(* Logix 5000 AddOnInstructionDefinition export Banner_WLS_Param_v4; software revision 33.00; part 2 of 3 *)
(* tags used below, declared in another part *)
   WLS : Banner_WLS_v4;
   Port_Data : Banner_IOL_Port_v4;
   Port : INT;   // Port Number that device is plugged into.
   Type : SINT;   // 0 = WLS27, 1 = WLS15, 2 = WLF
   Local_Control : DINT;
   Command_Being_Processed : BOOL;
   Update_Archive : BOOL;
   Index_Write_Inprocess : DINT;
   Index_Write_Control : DINT;
   Inprocess_Index : DINT;
   IndexR : DINT;   // Index keeping track of Reads in an array.
   S_Index : DINT;
   IndexW : DINT;   // Index keeping track of Writes in an array.
   LT_Index : DINT;
   IndexW2 : DINT;
   G_Index : DINT;
   IndexW3 : DINT;
(* Banner_WLS_Param_v4, continued *)

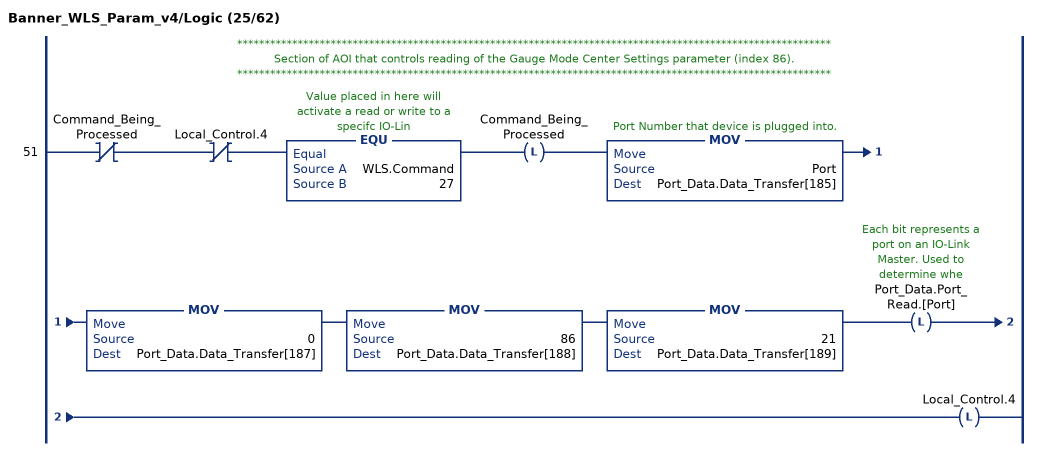
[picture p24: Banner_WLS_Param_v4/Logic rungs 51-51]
   // ************************************************************************************************************
   // Section of AOI that controls reading of the Gauge Mode Center Settings parameter (index 86).
   // ************************************************************************************************************
   51: XIO(Command_Being_Processed)XIO(Local_Control.4)EQU(WLS.Command,27)OTL(Command_Being_Processed)MOV(Port,Port_Data.Data_Transfer[185])MOV(0,Port_Data.Data_Transfer[187])MOV(86,Port_Data.Data_Transfer[188])MOV(21,Port_Data.Data_Transfer[189])OTL(Port_Data.Port_Read.[Port])OTL(Local_Control.4);
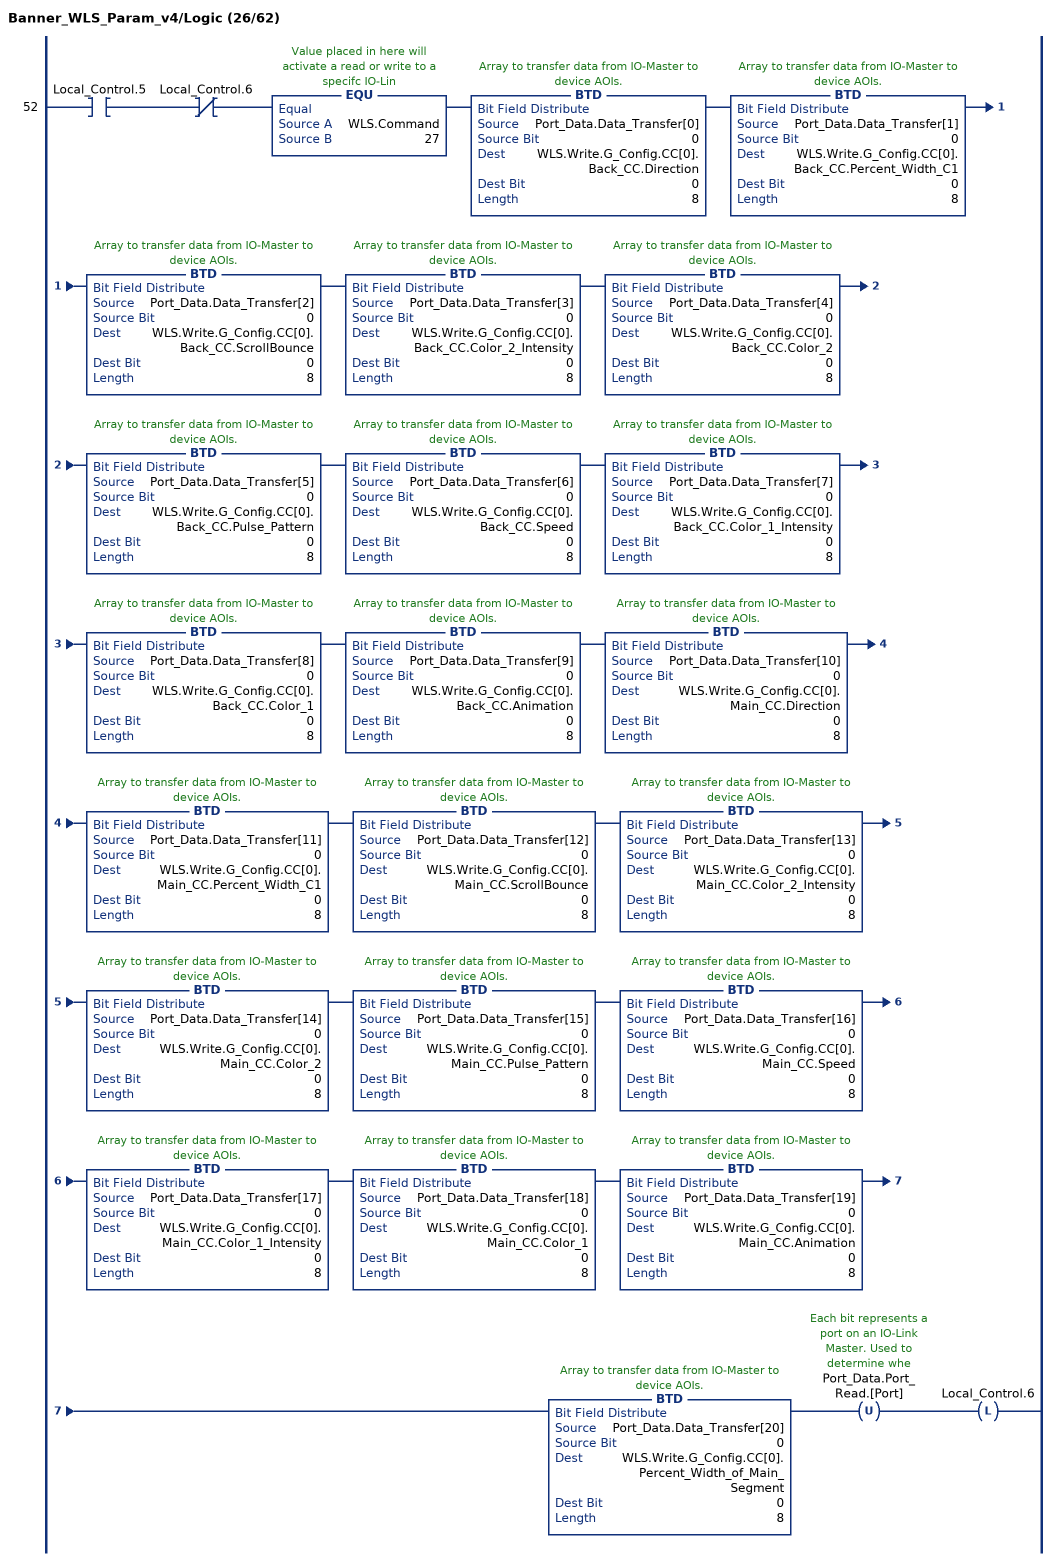
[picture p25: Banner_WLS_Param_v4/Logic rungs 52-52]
   52: XIC(Local_Control.5)XIO(Local_Control.6)EQU(WLS.Command,27)BTD(Port_Data.Data_Transfer[0],0,WLS.Write.G_Config.CC[0].Back_CC.Direction,0,8)BTD(Port_Data.Data_Transfer[1],0,WLS.Write.G_Config.CC[0].Back_CC.Percent_Width_C1,0,8)BTD(Port_Data.Data_Transfer[2],0,WLS.Write.G_Config.CC[0].Back_CC.ScrollBounce,0,8)BTD(Port_Data.Data_Transfer[3],0,WLS.Write.G_Config.CC[0].Back_CC.Color_2_Intensity,0,8)BTD(Port_Data.Data_Transfer[4],0,WLS.Write.G_Config.CC[0].Back_CC.Color_2,0,8)BTD(Port_Data.Data_Transfer[5],0,WLS.Write.G_Config.CC[0].Back_CC.Pulse_Pattern,0,8)BTD(Port_Data.Data_Transfer[6],0,WLS.Write.G_Config.CC[0].Back_CC.Speed,0,8)BTD(Port_Data.Data_Transfer[7],0,WLS.Write.G_Config.CC[0].Back_CC.Color_1_Intensity,0,8)BTD(Port_Data.Data_Transfer[8],0,WLS.Write.G_Config.CC[0].Back_CC.Color_1,0,8)BTD(Port_Data.Data_Transfer[9],0,WLS.Write.G_Config.CC[0].Back_CC.Animation,0,8)BTD(Port_Data.Data_Transfer[10],0,WLS.Write.G_Config.CC[0].Main_CC.Direction,0,8)BTD(Port_Data.Data_Transfer[11],0,WLS.Write.G_Config.CC[0].Main_CC.Percent_Width_C1,0,8)BTD(Port_Data.Data_Transfer[12],0,WLS.Write.G_Config.CC[0].Main_CC.ScrollBounce,0,8)BTD(Port_Data.Data_Transfer[13],0,WLS.Write.G_Config.CC[0].Main_CC.Color_2_Intensity,0,8)BTD(Port_Data.Data_Transfer[14],0,WLS.Write.G_Config.CC[0].Main_CC.Color_2,0,8)BTD(Port_Data.Data_Transfer[15],0,WLS.Write.G_Config.CC[0].Main_CC.Pulse_Pattern,0,8)BTD(Port_Data.Data_Transfer[16],0,WLS.Write.G_Config.CC[0].Main_CC.Speed,0,8)BTD(Port_Data.Data_Transfer[17],0,WLS.Write.G_Config.CC[0].Main_CC.Color_1_Intensity,0,8)BTD(Port_Data.Data_Transfer[18],0,WLS.Write.G_Config.CC[0].Main_CC.Color_1,0,8)BTD(Port_Data.Data_Transfer[19],0,WLS.Write.G_Config.CC[0].Main_CC.Animation,0,8)BTD(Port_Data.Data_Transfer[20],0,WLS.Write.G_Config.CC[0].Percent_Width_of_Main_Segment,0,8)OTU(Port_Data.Port_Read.[Port])OTL(Local_Control.6);
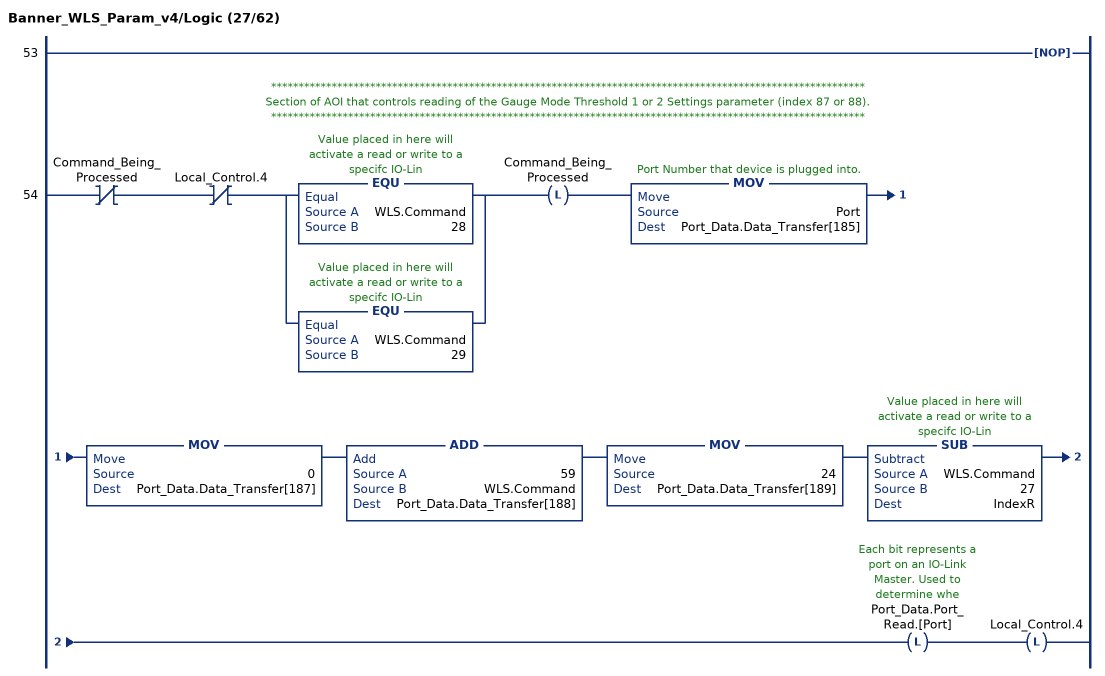
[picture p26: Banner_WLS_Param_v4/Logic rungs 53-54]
   53: NOP();
   // ************************************************************************************************************
   // Section of AOI that controls reading of the Gauge Mode Threshold 1 or 2 Settings parameter (index 87 or 88).
   // ************************************************************************************************************
   54: XIO(Command_Being_Processed)XIO(Local_Control.4)[EQU(WLS.Command,28) ,EQU(WLS.Command,29) ]OTL(Command_Being_Processed)MOV(Port,Port_Data.Data_Transfer[185])MOV(0,Port_Data.Data_Transfer[187])ADD(59,WLS.Command,Port_Data.Data_Transfer[188])MOV(24,Port_Data.Data_Transfer[189])SUB(WLS.Command,27,IndexR)OTL(Port_Data.Port_Read.[Port])OTL(Local_Control.4);
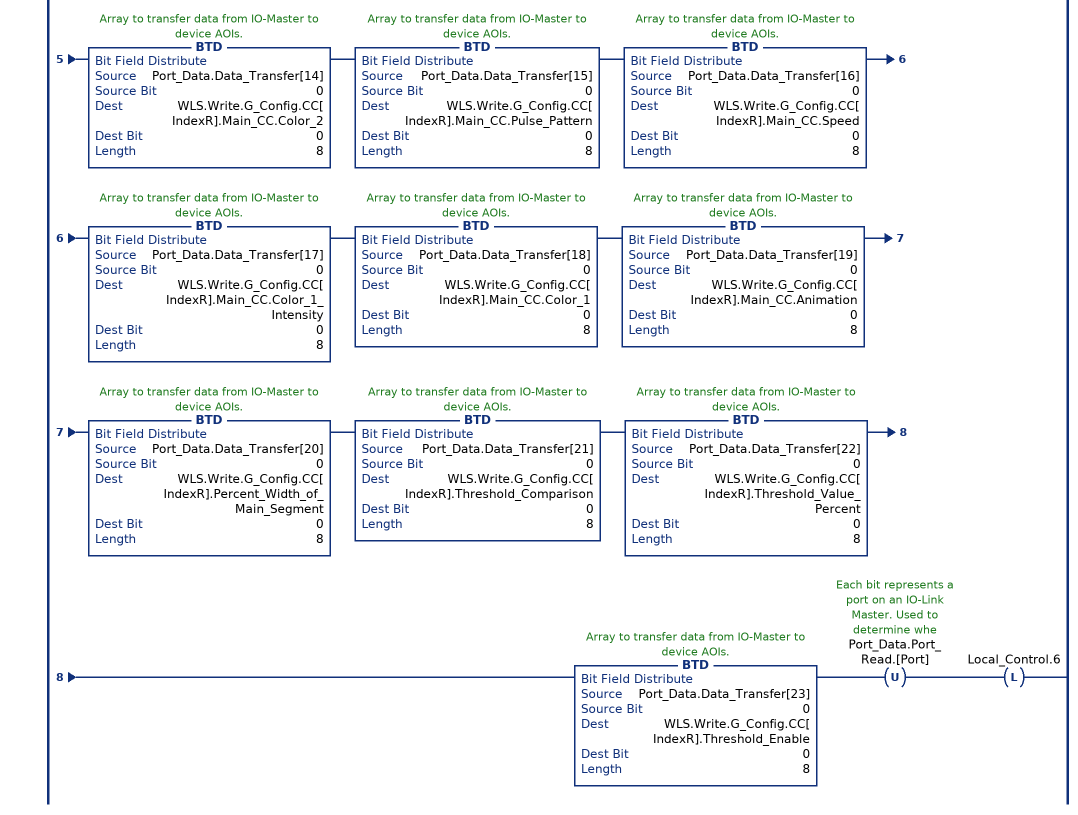
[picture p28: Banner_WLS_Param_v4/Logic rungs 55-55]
   55: XIC(Local_Control.5)XIO(Local_Control.6)[EQU(WLS.Command,28) ,EQU(WLS.Command,29) ]BTD(Port_Data.Data_Transfer[0],0,WLS.Write.G_Config.CC[IndexR].Back_CC.Direction,0,8)BTD(Port_Data.Data_Transfer[1],0,WLS.Write.G_Config.CC[IndexR].Back_CC.Percent_Width_C1,0,8)BTD(Port_Data.Data_Transfer[2],0,WLS.Write.G_Config.CC[IndexR].Back_CC.ScrollBounce,0,8)BTD(Port_Data.Data_Transfer[3],0,WLS.Write.G_Config.CC[IndexR].Back_CC.Color_2_Intensity,0,8)BTD(Port_Data.Data_Transfer[4],0,WLS.Write.G_Config.CC[IndexR].Back_CC.Color_2,0,8)BTD(Port_Data.Data_Transfer[5],0,WLS.Write.G_Config.CC[IndexR].Back_CC.Pulse_Pattern,0,8)BTD(Port_Data.Data_Transfer[6],0,WLS.Write.G_Config.CC[IndexR].Back_CC.Speed,0,8)BTD(Port_Data.Data_Transfer[7],0,WLS.Write.G_Config.CC[IndexR].Back_CC.Color_1_Intensity,0,8)BTD(Port_Data.Data_Transfer[8],0,WLS.Write.G_Config.CC[IndexR].Back_CC.Color_1,0,8)BTD(Port_Data.Data_Transfer[9],0,WLS.Write.G_Config.CC[IndexR].Back_CC.Animation,0,8)BTD(Port_Data.Data_Transfer[10],0,WLS.Write.G_Config.CC[IndexR].Main_CC.Direction,0,8)BTD(Port_Data.Data_Transfer[11],0,WLS.Write.G_Config.CC[IndexR].Main_CC.Percent_Width_C1,0,8)BTD(Port_Data.Data_Transfer[12],0,WLS.Write.G_Config.CC[IndexR].Main_CC.ScrollBounce,0,8)BTD(Port_Data.Data_Transfer[13],0,WLS.Write.G_Config.CC[IndexR].Main_CC.Color_2_Intensity,0,8)BTD(Port_Data.Data_Transfer[14],0,WLS.Write.G_Config.CC[IndexR].Main_CC.Color_2,0,8)BTD(Port_Data.Data_Transfer[15],0,WLS.Write.G_Config.CC[IndexR].Main_CC.Pulse_Pattern,0,8)BTD(Port_Data.Data_Transfer[16],0,WLS.Write.G_Config.CC[IndexR].Main_CC.Speed,0,8)BTD(Port_Data.Data_Transfer[17],0,WLS.Write.G_Config.CC[IndexR].Main_CC.Color_1_Intensity,0,8)BTD(Port_Data.Data_Transfer[18],0,WLS.Write.G_Config.CC[IndexR].Main_CC.Color_1,0,8)BTD(Port_Data.Data_Transfer[19],0,WLS.Write.G_Config.CC[IndexR].Main_CC.Animation,0,8)BTD(Port_Data.Data_Transfer[20],0,WLS.Write.G_Config.CC[IndexR].Percent_Width_of_Main_Segment,0,8)BTD(Port_Data.Data_Transfer[21],0,WLS.Write.G_Config.CC[IndexR].Threshold_Comparison,0,8)BTD(Port_Data.Data_Transfer[22],0,WLS.Write.G_Config.CC[IndexR].Threshold_Value_Percent,0,8)BTD(Port_Data.Data_Transfer[23],0,WLS.Write.G_Config.CC[IndexR].Threshold_Enable,0,8)OTU(Port_Data.Port_Read.[Port])OTL(Local_Control.6);
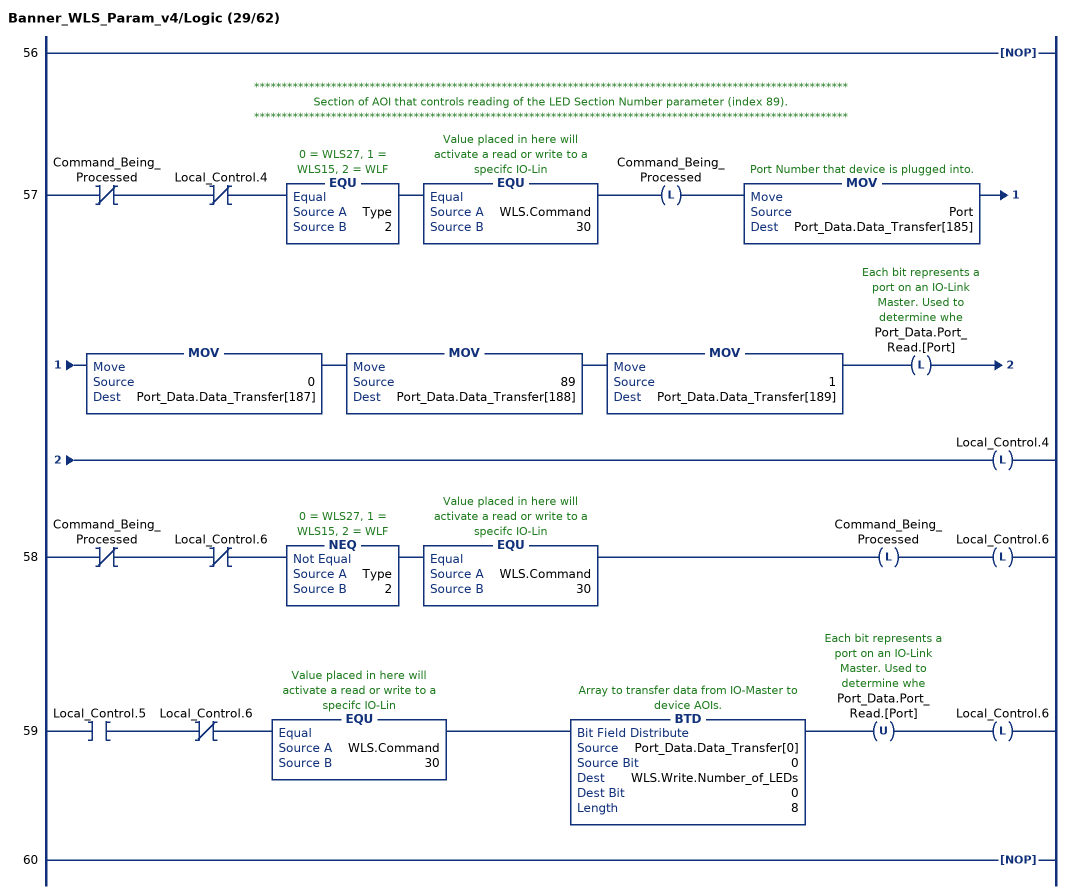
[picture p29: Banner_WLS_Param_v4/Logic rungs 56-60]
   56: NOP();
   // ************************************************************************************************************
   // Section of AOI that controls reading of the LED Section Number parameter (index 89).
   // ************************************************************************************************************
   57: XIO(Command_Being_Processed)XIO(Local_Control.4)EQU(Type,2)EQU(WLS.Command,30)OTL(Command_Being_Processed)MOV(Port,Port_Data.Data_Transfer[185])MOV(0,Port_Data.Data_Transfer[187])MOV(89,Port_Data.Data_Transfer[188])MOV(1,Port_Data.Data_Transfer[189])OTL(Port_Data.Port_Read.[Port])OTL(Local_Control.4);
   58: XIO(Command_Being_Processed)XIO(Local_Control.6)NEQ(Type,2)EQU(WLS.Command,30)OTL(Command_Being_Processed)OTL(Local_Control.6);
   59: XIC(Local_Control.5)XIO(Local_Control.6)EQU(WLS.Command,30)BTD(Port_Data.Data_Transfer[0],0,WLS.Write.Number_of_LEDs,0,8)OTU(Port_Data.Port_Read.[Port])OTL(Local_Control.6);
   60: NOP();
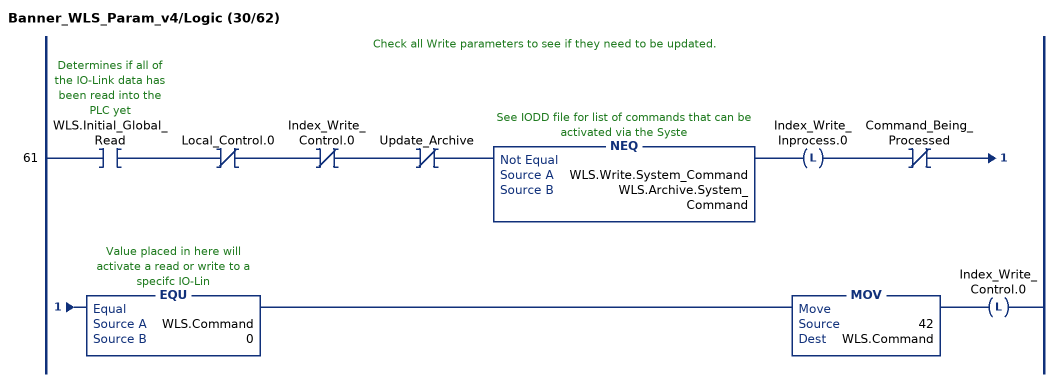
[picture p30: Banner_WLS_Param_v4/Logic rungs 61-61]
   // Check all Write parameters to see if they need to be updated.
   61: XIC(WLS.Initial_Global_Read)XIO(Local_Control.0)XIO(Index_Write_Control.0)XIO(Update_Archive)NEQ(WLS.Write.System_Command,WLS.Archive.System_Command)OTL(Index_Write_Inprocess.0)XIO(Command_Being_Processed)EQU(WLS.Command,0)MOV(42,WLS.Command)OTL(Index_Write_Control.0);
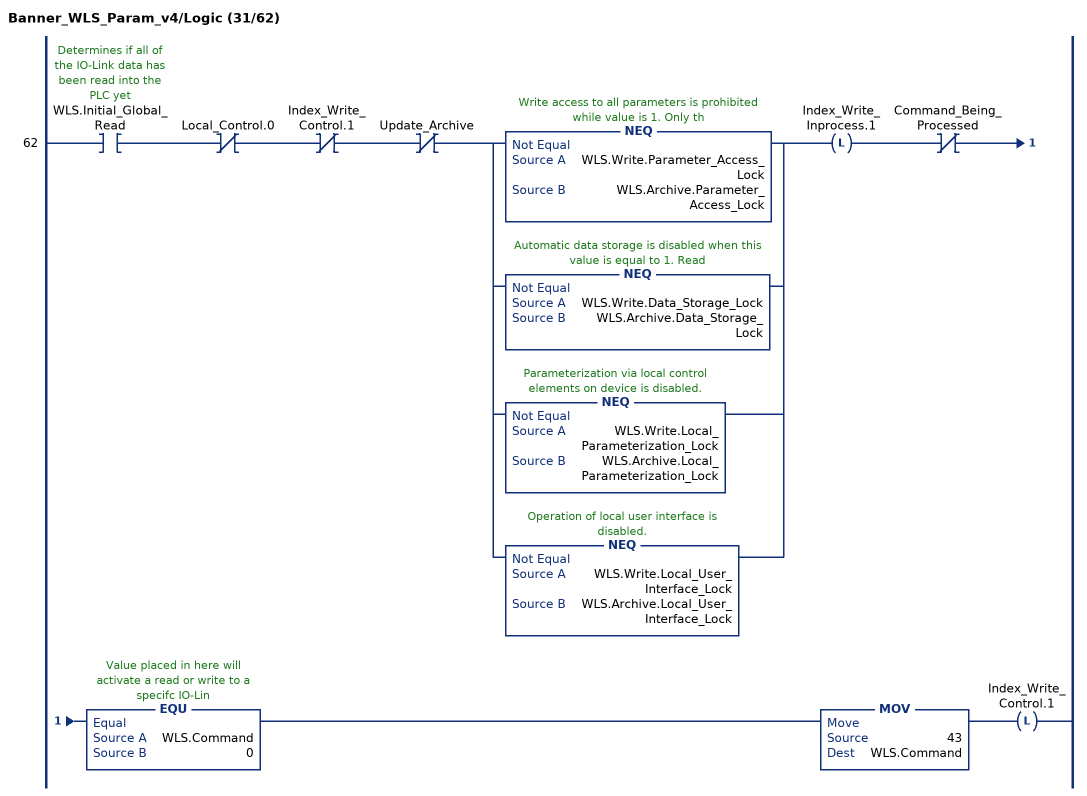
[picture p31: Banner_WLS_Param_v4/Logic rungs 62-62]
   62: XIC(WLS.Initial_Global_Read)XIO(Local_Control.0)XIO(Index_Write_Control.1)XIO(Update_Archive)[NEQ(WLS.Write.Parameter_Access_Lock,WLS.Archive.Parameter_Access_Lock) ,NEQ(WLS.Write.Data_Storage_Lock,WLS.Archive.Data_Storage_Lock) ,NEQ(WLS.Write.Local_Parameterization_Lock,WLS.Archive.Local_Parameterization_Lock) ,NEQ(WLS.Write.Local_User_Interface_Lock,WLS.Archive.Local_User_Interface_Lock) ]OTL(Index_Write_Inprocess.1)XIO(Command_Being_Processed)EQU(WLS.Command,0)MOV(43,WLS.Command)OTL(Index_Write_Control.1);
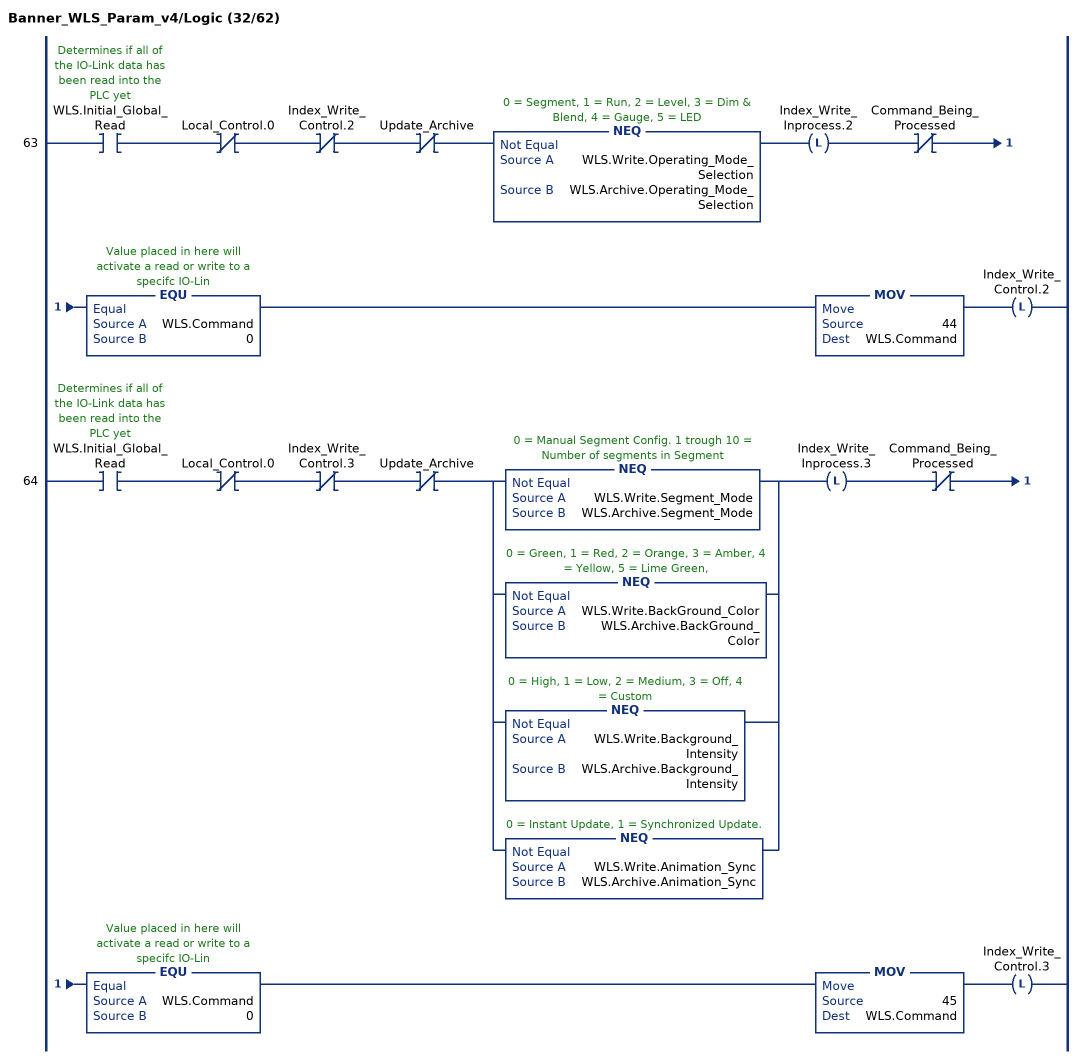
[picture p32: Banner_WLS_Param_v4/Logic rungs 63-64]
   63: XIC(WLS.Initial_Global_Read)XIO(Local_Control.0)XIO(Index_Write_Control.2)XIO(Update_Archive)NEQ(WLS.Write.Operating_Mode_Selection,WLS.Archive.Operating_Mode_Selection)OTL(Index_Write_Inprocess.2)XIO(Command_Being_Processed)EQU(WLS.Command,0)MOV(44,WLS.Command)OTL(Index_Write_Control.2);
   64: XIC(WLS.Initial_Global_Read)XIO(Local_Control.0)XIO(Index_Write_Control.3)XIO(Update_Archive)[NEQ(WLS.Write.Segment_Mode,WLS.Archive.Segment_Mode) ,NEQ(WLS.Write.BackGround_Color,WLS.Archive.BackGround_Color) ,NEQ(WLS.Write.Background_Intensity,WLS.Archive.Background_Intensity) ,NEQ(WLS.Write.Animation_Sync,WLS.Archive.Animation_Sync) ]OTL(Index_Write_Inprocess.3)XIO(Command_Being_Processed)EQU(WLS.Command,0)MOV(45,WLS.Command)OTL(Index_Write_Control.3);
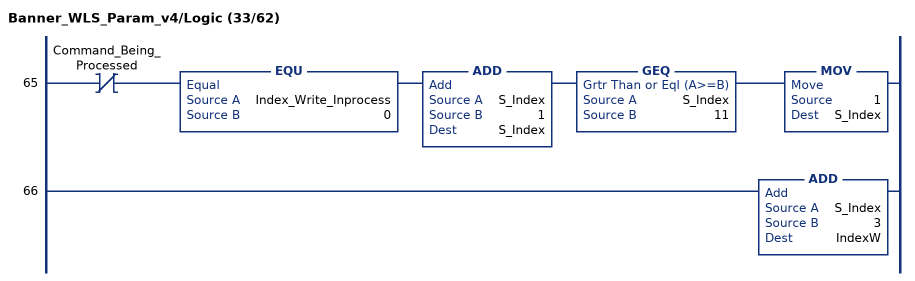
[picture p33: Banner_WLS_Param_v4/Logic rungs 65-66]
   65: XIO(Command_Being_Processed)EQU(Index_Write_Inprocess,0)ADD(S_Index,1,S_Index)GEQ(S_Index,11)MOV(1,S_Index);
   66: ADD(S_Index,3,IndexW);
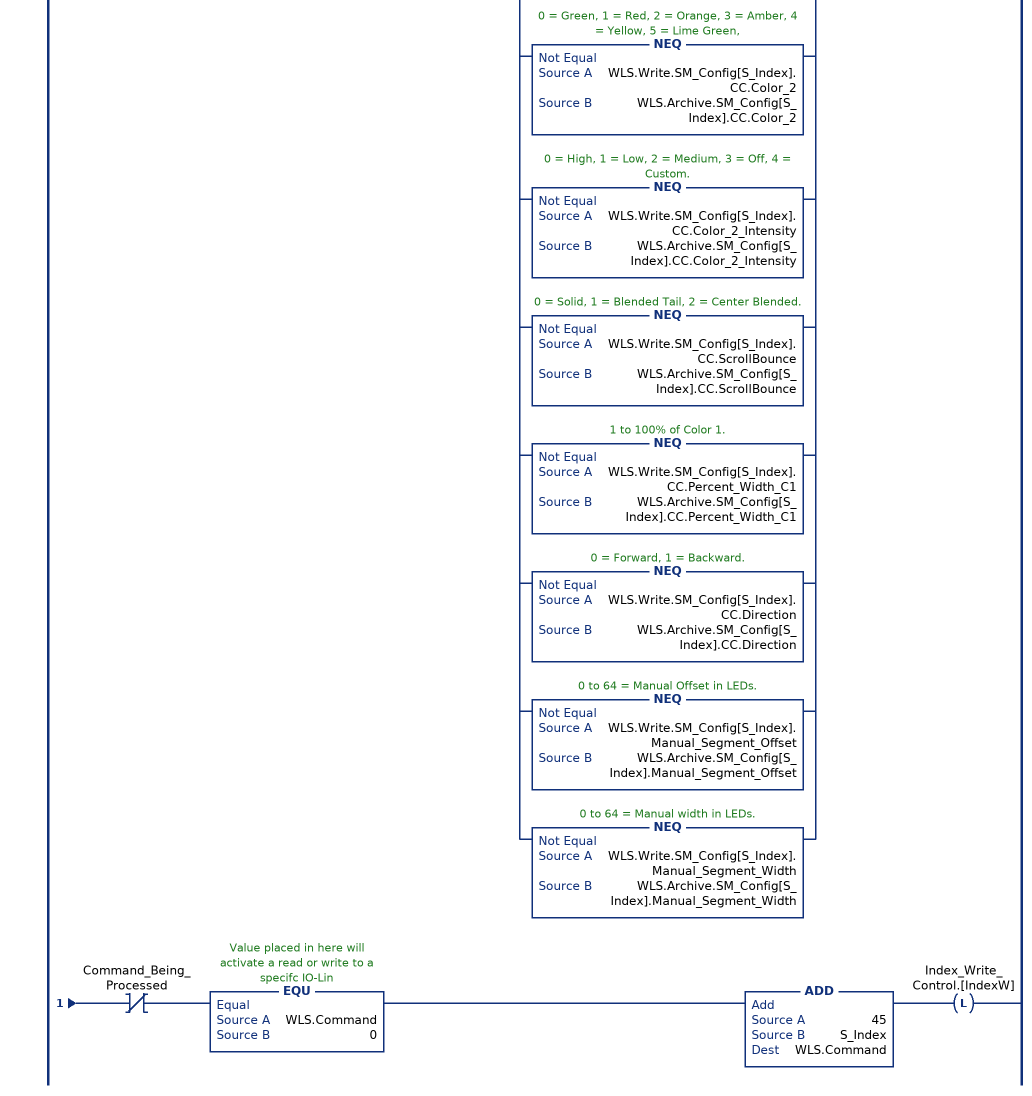
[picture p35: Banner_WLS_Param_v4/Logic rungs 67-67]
   67: XIC(WLS.Initial_Global_Read)XIO(Local_Control.0)XIO(Index_Write_Control.[IndexW])XIO(Update_Archive)[NEQ(WLS.Write.SM_Config[S_Index].Basic_Color,WLS.Archive.SM_Config[S_Index].Basic_Color) ,NEQ(WLS.Write.SM_Config[S_Index].Basic_Flash_Rate,WLS.Archive.SM_Config[S_Index].Basic_Flash_Rate) ,NEQ(WLS.Write.SM_Config[S_Index].CC.Animation,WLS.Archive.SM_Config[S_Index].CC.Animation) ,NEQ(WLS.Write.SM_Config[S_Index].CC.Color_1,WLS.Archive.SM_Config[S_Index].CC.Color_1) ,NEQ(WLS.Write.SM_Config[S_Index].CC.Color_1_Intensity,WLS.Archive.SM_Config[S_Index].CC.Color_1_Intensity) ,NEQ(WLS.Write.SM_Config[S_Index].CC.Speed,WLS.Archive.SM_Config[S_Index].CC.Speed) ,NEQ(WLS.Write.SM_Config[S_Index].CC.Pulse_Pattern,WLS.Archive.SM_Config[S_Index].CC.Pulse_Pattern) ,NEQ(WLS.Write.SM_Config[S_Index].CC.Color_2,WLS.Archive.SM_Config[S_Index].CC.Color_2) ,NEQ(WLS.Write.SM_Config[S_Index].CC.Color_2_Intensity,WLS.Archive.SM_Config[S_Index].CC.Color_2_Intensity) ,NEQ(WLS.Write.SM_Config[S_Index].CC.ScrollBounce,WLS.Archive.SM_Config[S_Index].CC.ScrollBounce) ,NEQ(WLS.Write.SM_Config[S_Index].CC.Percent_Width_C1,WLS.Archive.SM_Config[S_Index].CC.Percent_Width_C1) ,NEQ(WLS.Write.SM_Config[S_Index].CC.Direction,WLS.Archive.SM_Config[S_Index].CC.Direction) ,NEQ(WLS.Write.SM_Config[S_Index].Manual_Segment_Offset,WLS.Archive.SM_Config[S_Index].Manual_Segment_Offset) ,NEQ(WLS.Write.SM_Config[S_Index].Manual_Segment_Width,WLS.Archive.SM_Config[S_Index].Manual_Segment_Width) ]OTL(Index_Write_Inprocess.[IndexW])XIO(Command_Being_Processed)EQU(WLS.Command,0)ADD(45,S_Index,WLS.Command)OTL(Index_Write_Control.[IndexW]);
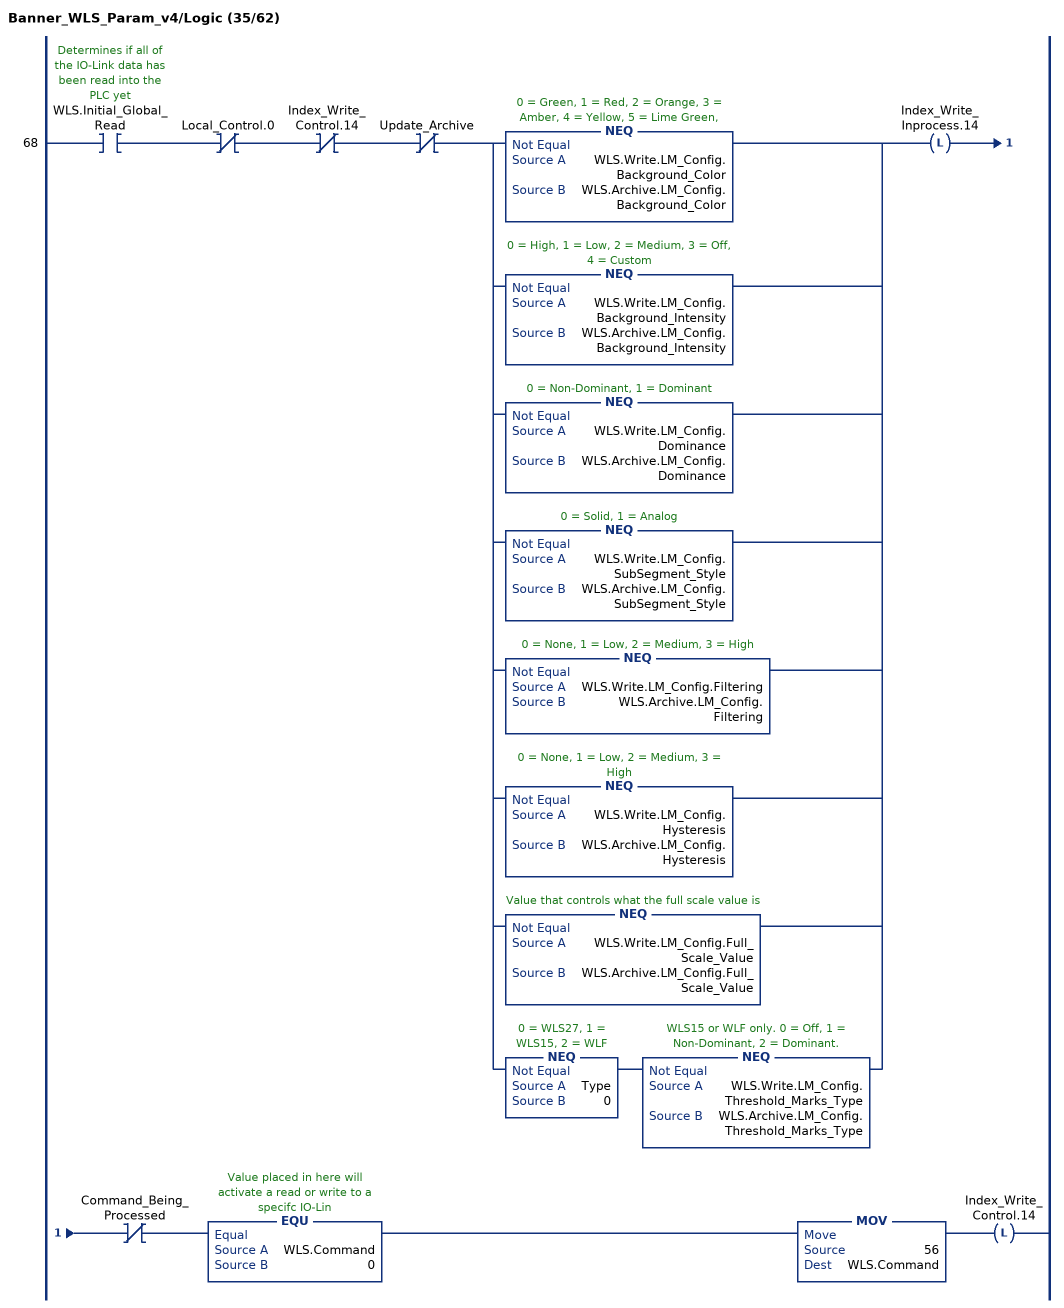
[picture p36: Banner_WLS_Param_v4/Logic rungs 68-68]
   68: XIC(WLS.Initial_Global_Read)XIO(Local_Control.0)XIO(Index_Write_Control.14)XIO(Update_Archive)[NEQ(WLS.Write.LM_Config.Background_Color,WLS.Archive.LM_Config.Background_Color) ,NEQ(WLS.Write.LM_Config.Background_Intensity,WLS.Archive.LM_Config.Background_Intensity) ,NEQ(WLS.Write.LM_Config.Dominance,WLS.Archive.LM_Config.Dominance) ,NEQ(WLS.Write.LM_Config.SubSegment_Style,WLS.Archive.LM_Config.SubSegment_Style) ,NEQ(WLS.Write.LM_Config.Filtering,WLS.Archive.LM_Config.Filtering) ,NEQ(WLS.Write.LM_Config.Hysteresis,WLS.Archive.LM_Config.Hysteresis) ,NEQ(WLS.Write.LM_Config.Full_Scale_Value,WLS.Archive.LM_Config.Full_Scale_Value) ,NEQ(Type,0) NEQ(WLS.Write.LM_Config.Threshold_Marks_Type,WLS.Archive.LM_Config.Threshold_Marks_Type) ]OTL(Index_Write_Inprocess.14)XIO(Command_Being_Processed)EQU(WLS.Command,0)MOV(56,WLS.Command)OTL(Index_Write_Control.14);
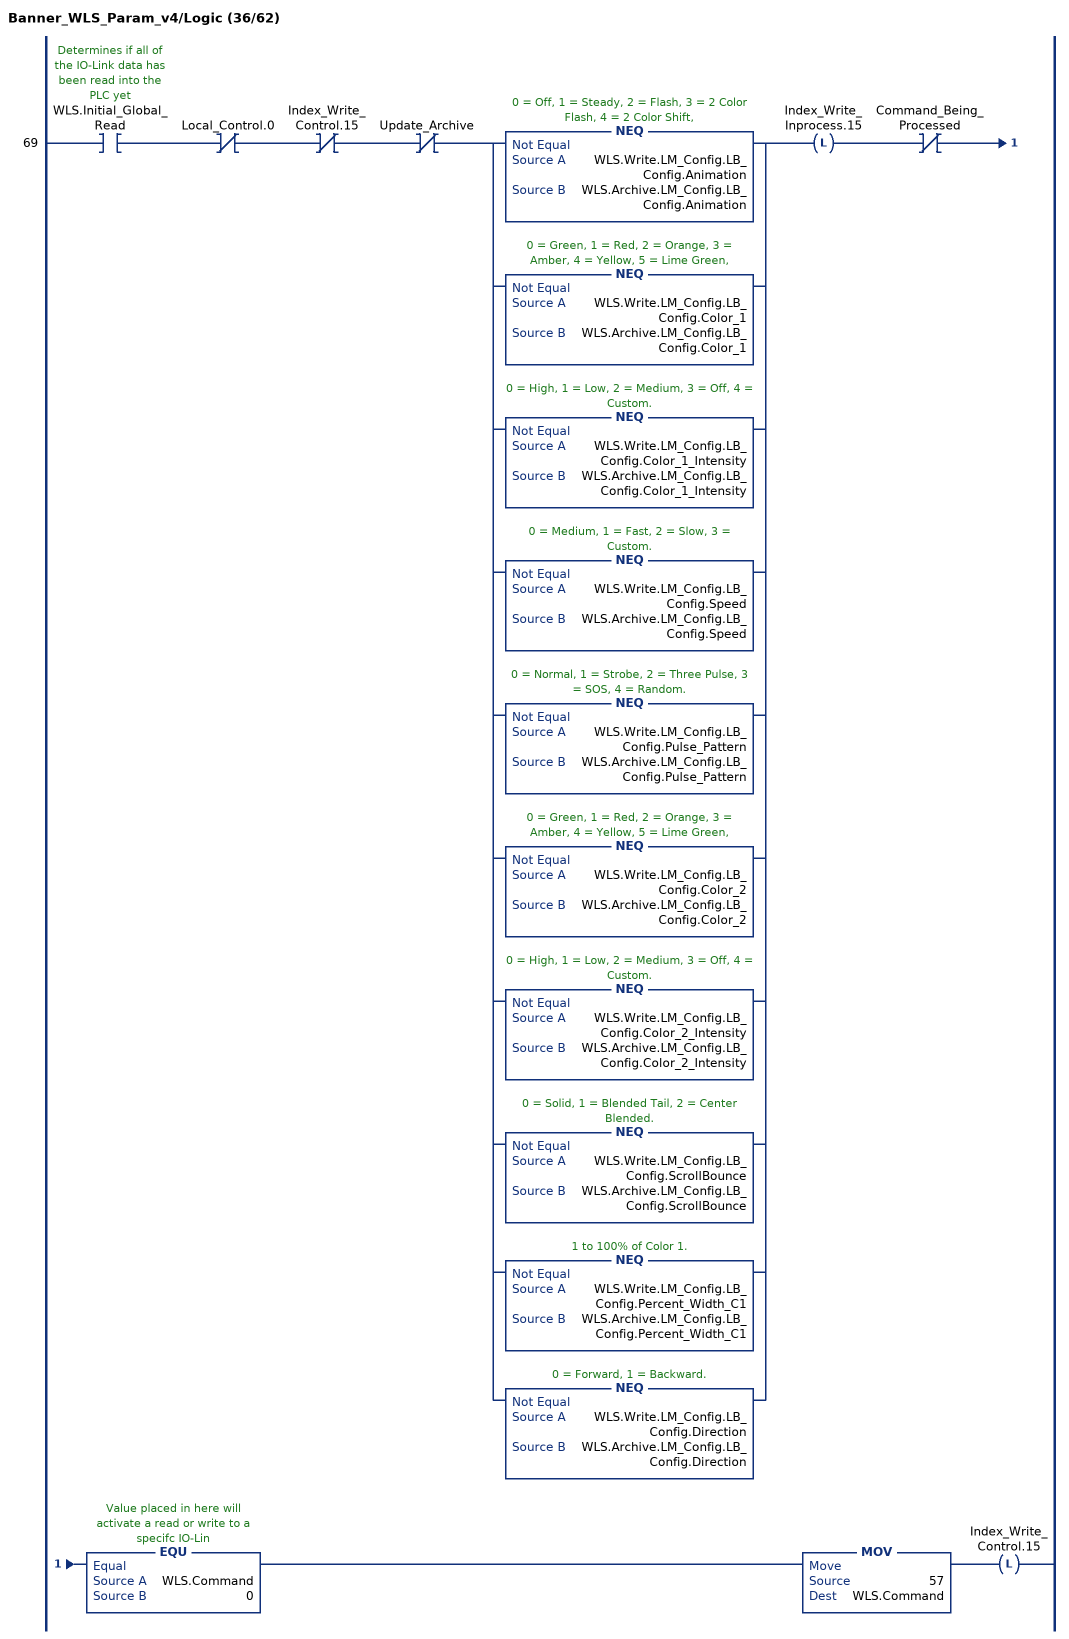
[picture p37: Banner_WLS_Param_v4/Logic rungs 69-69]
   69: XIC(WLS.Initial_Global_Read)XIO(Local_Control.0)XIO(Index_Write_Control.15)XIO(Update_Archive)[NEQ(WLS.Write.LM_Config.LB_Config.Animation,WLS.Archive.LM_Config.LB_Config.Animation) ,NEQ(WLS.Write.LM_Config.LB_Config.Color_1,WLS.Archive.LM_Config.LB_Config.Color_1) ,NEQ(WLS.Write.LM_Config.LB_Config.Color_1_Intensity,WLS.Archive.LM_Config.LB_Config.Color_1_Intensity) ,NEQ(WLS.Write.LM_Config.LB_Config.Speed,WLS.Archive.LM_Config.LB_Config.Speed) ,NEQ(WLS.Write.LM_Config.LB_Config.Pulse_Pattern,WLS.Archive.LM_Config.LB_Config.Pulse_Pattern) ,NEQ(WLS.Write.LM_Config.LB_Config.Color_2,WLS.Archive.LM_Config.LB_Config.Color_2) ,NEQ(WLS.Write.LM_Config.LB_Config.Color_2_Intensity,WLS.Archive.LM_Config.LB_Config.Color_2_Intensity) ,NEQ(WLS.Write.LM_Config.LB_Config.ScrollBounce,WLS.Archive.LM_Config.LB_Config.ScrollBounce) ,NEQ(WLS.Write.LM_Config.LB_Config.Percent_Width_C1,WLS.Archive.LM_Config.LB_Config.Percent_Width_C1) ,NEQ(WLS.Write.LM_Config.LB_Config.Direction,WLS.Archive.LM_Config.LB_Config.Direction) ]OTL(Index_Write_Inprocess.15)XIO(Command_Being_Processed)EQU(WLS.Command,0)MOV(57,WLS.Command)OTL(Index_Write_Control.15);
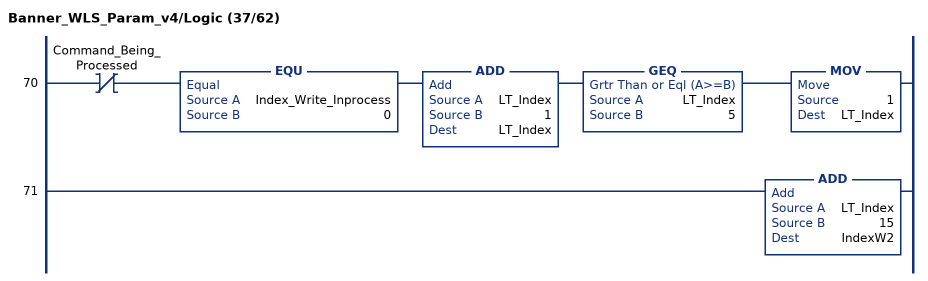
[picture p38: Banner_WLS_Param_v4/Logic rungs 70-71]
   70: XIO(Command_Being_Processed)EQU(Index_Write_Inprocess,0)ADD(LT_Index,1,LT_Index)GEQ(LT_Index,5)MOV(1,LT_Index);
   71: ADD(LT_Index,15,IndexW2);
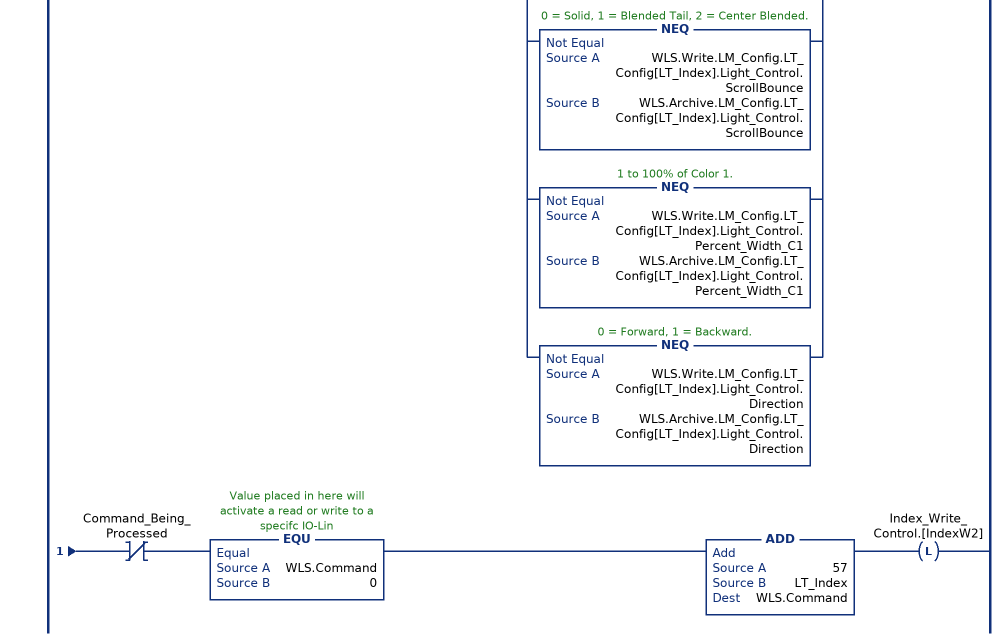
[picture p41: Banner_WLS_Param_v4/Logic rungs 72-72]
   72: XIC(WLS.Initial_Global_Read)XIO(Local_Control.0)XIO(Index_Write_Control.[IndexW2])XIO(Update_Archive)[NEQ(WLS.Write.LM_Config.LT_Config[LT_Index].Threshold_Enable,WLS.Archive.LM_Config.LT_Config[LT_Index].Threshold_Enable) ,NEQ(WLS.Write.LM_Config.LT_Config[LT_Index].Threshold_Value,WLS.Archive.LM_Config.LT_Config[LT_Index].Threshold_Value) ,NEQ(WLS.Write.LM_Config.LT_Config[LT_Index].Threshold_Comparison,WLS.Archive.LM_Config.LT_Config[LT_Index].Threshold_Comparison) ,NEQ(WLS.Write.LM_Config.LT_Config[LT_Index].Threshold_Override,WLS.Archive.LM_Config.LT_Config[LT_Index].Threshold_Override) ,NEQ(WLS.Write.LM_Config.LT_Config[LT_Index].Light_Control.Animation,WLS.Archive.LM_Config.LT_Config[LT_Index].Light_Control.Animation) ,NEQ(WLS.Write.LM_Config.LT_Config[LT_Index].Light_Control.Color_1,WLS.Archive.LM_Config.LT_Config[LT_Index].Light_Control.Color_1) ,NEQ(WLS.Write.LM_Config.LT_Config[LT_Index].Light_Control.Color_1_Intensity,WLS.Archive.LM_Config.LT_Config[LT_Index].Light_Control.Color_1_Intensity) ,NEQ(WLS.Write.LM_Config.LT_Config[LT_Index].Light_Control.Speed,WLS.Archive.LM_Config.LT_Config[LT_Index].Light_Control.Speed) ,NEQ(WLS.Write.LM_Config.LT_Config[LT_Index].Light_Control.Pulse_Pattern,WLS.Archive.LM_Config.LT_Config[LT_Index].Light_Control.Pulse_Pattern) ,NEQ(WLS.Write.LM_Config.LT_Config[LT_Index].Light_Control.Color_2,WLS.Archive.LM_Config.LT_Config[LT_Index].Light_Control.Color_2) ,NEQ(WLS.Write.LM_Config.LT_Config[LT_Index].Light_Control.Color_2_Intensity,WLS.Archive.LM_Config.LT_Config[LT_Index].Light_Control.Color_2_Intensity) ,NEQ(WLS.Write.LM_Config.LT_Config[LT_Index].Light_Control.ScrollBounce,WLS.Archive.LM_Config.LT_Config[LT_Index].Light_Control.ScrollBounce) ,NEQ(WLS.Write.LM_Config.LT_Config[LT_Index].Light_Control.Percent_Width_C1,WLS.Archive.LM_Config.LT_Config[LT_Index].Light_Control.Percent_Width_C1) ,NEQ(WLS.Write.LM_Config.LT_Config[LT_Index].Light_Control.Direction,WLS.Archive.LM_Config.LT_Config[LT_Index].Light_Control.Direction) ]OTL(Index_Write_Inprocess.[IndexW2])XIO(Command_Being_Processed)EQU(WLS.Command,0)ADD(57,LT_Index,WLS.Command)OTL(Index_Write_Control.[IndexW2]);
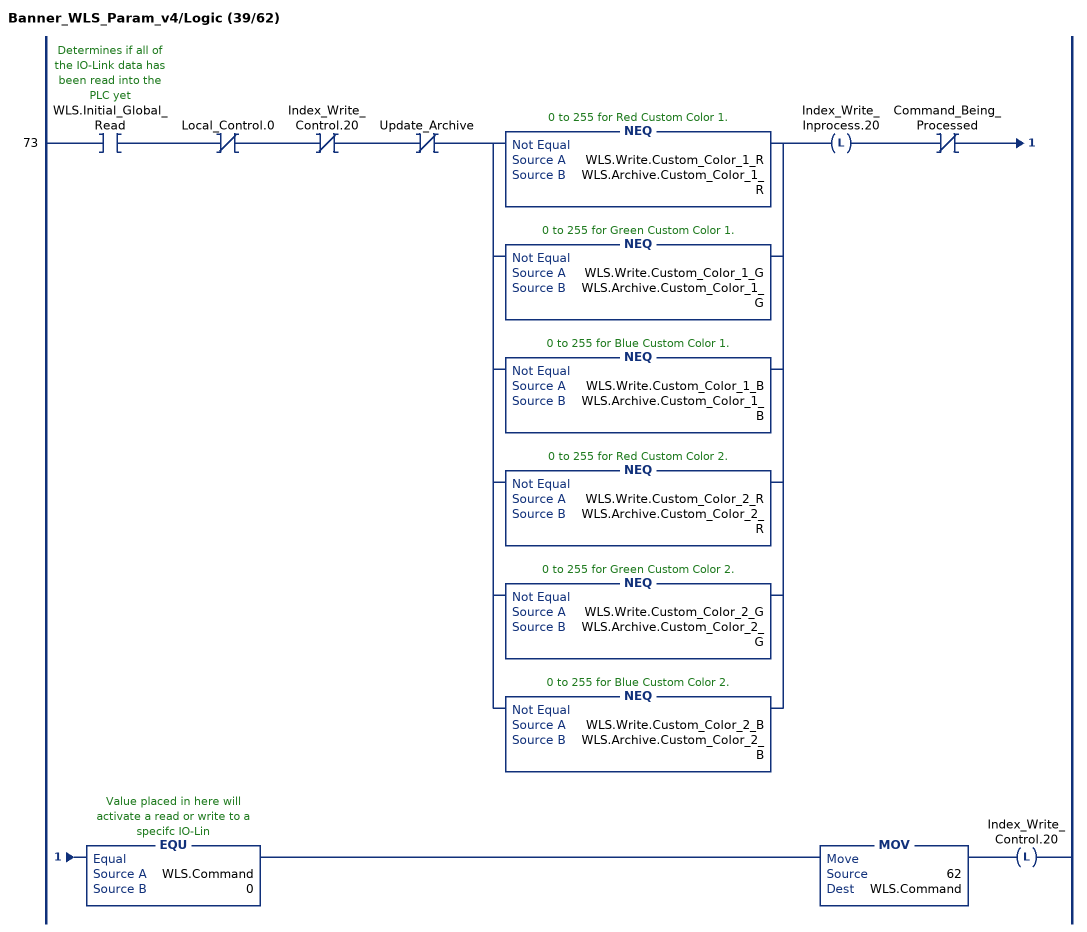
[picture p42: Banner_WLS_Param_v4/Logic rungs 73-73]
   73: XIC(WLS.Initial_Global_Read)XIO(Local_Control.0)XIO(Index_Write_Control.20)XIO(Update_Archive)[NEQ(WLS.Write.Custom_Color_1_R,WLS.Archive.Custom_Color_1_R) ,NEQ(WLS.Write.Custom_Color_1_G,WLS.Archive.Custom_Color_1_G) ,NEQ(WLS.Write.Custom_Color_1_B,WLS.Archive.Custom_Color_1_B) ,NEQ(WLS.Write.Custom_Color_2_R,WLS.Archive.Custom_Color_2_R) ,NEQ(WLS.Write.Custom_Color_2_G,WLS.Archive.Custom_Color_2_G) ,NEQ(WLS.Write.Custom_Color_2_B,WLS.Archive.Custom_Color_2_B) ]OTL(Index_Write_Inprocess.20)XIO(Command_Being_Processed)EQU(WLS.Command,0)MOV(62,WLS.Command)OTL(Index_Write_Control.20);
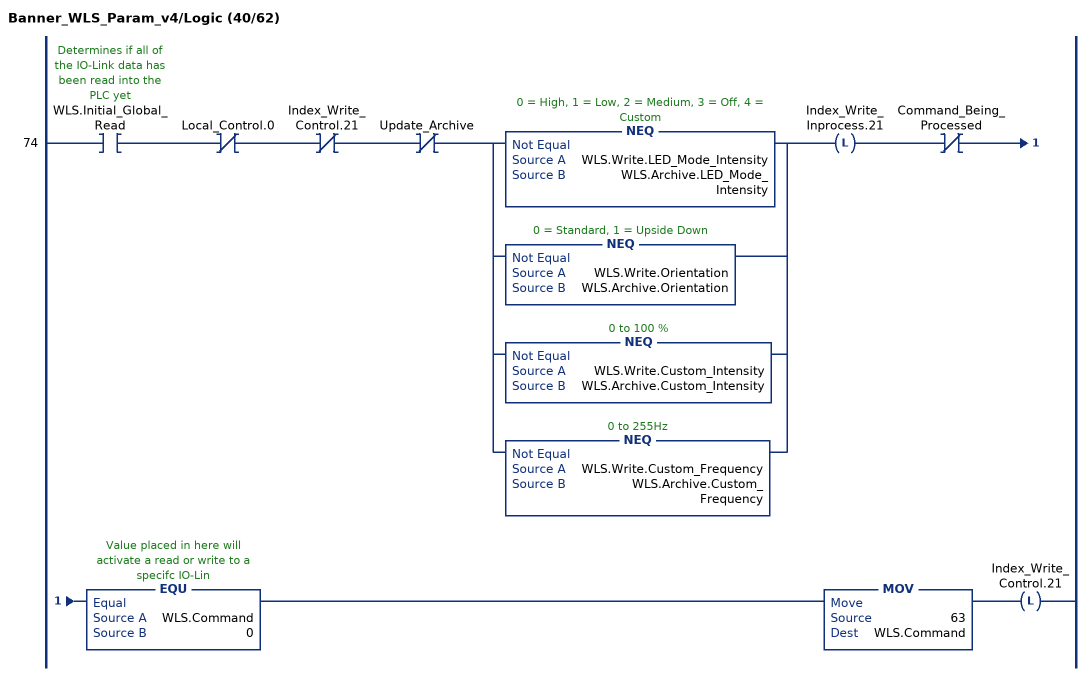
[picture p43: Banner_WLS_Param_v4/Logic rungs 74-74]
   74: XIC(WLS.Initial_Global_Read)XIO(Local_Control.0)XIO(Index_Write_Control.21)XIO(Update_Archive)[NEQ(WLS.Write.LED_Mode_Intensity,WLS.Archive.LED_Mode_Intensity) ,NEQ(WLS.Write.Orientation,WLS.Archive.Orientation) ,NEQ(WLS.Write.Custom_Intensity,WLS.Archive.Custom_Intensity) ,NEQ(WLS.Write.Custom_Frequency,WLS.Archive.Custom_Frequency) ]OTL(Index_Write_Inprocess.21)XIO(Command_Being_Processed)EQU(WLS.Command,0)MOV(63,WLS.Command)OTL(Index_Write_Control.21);
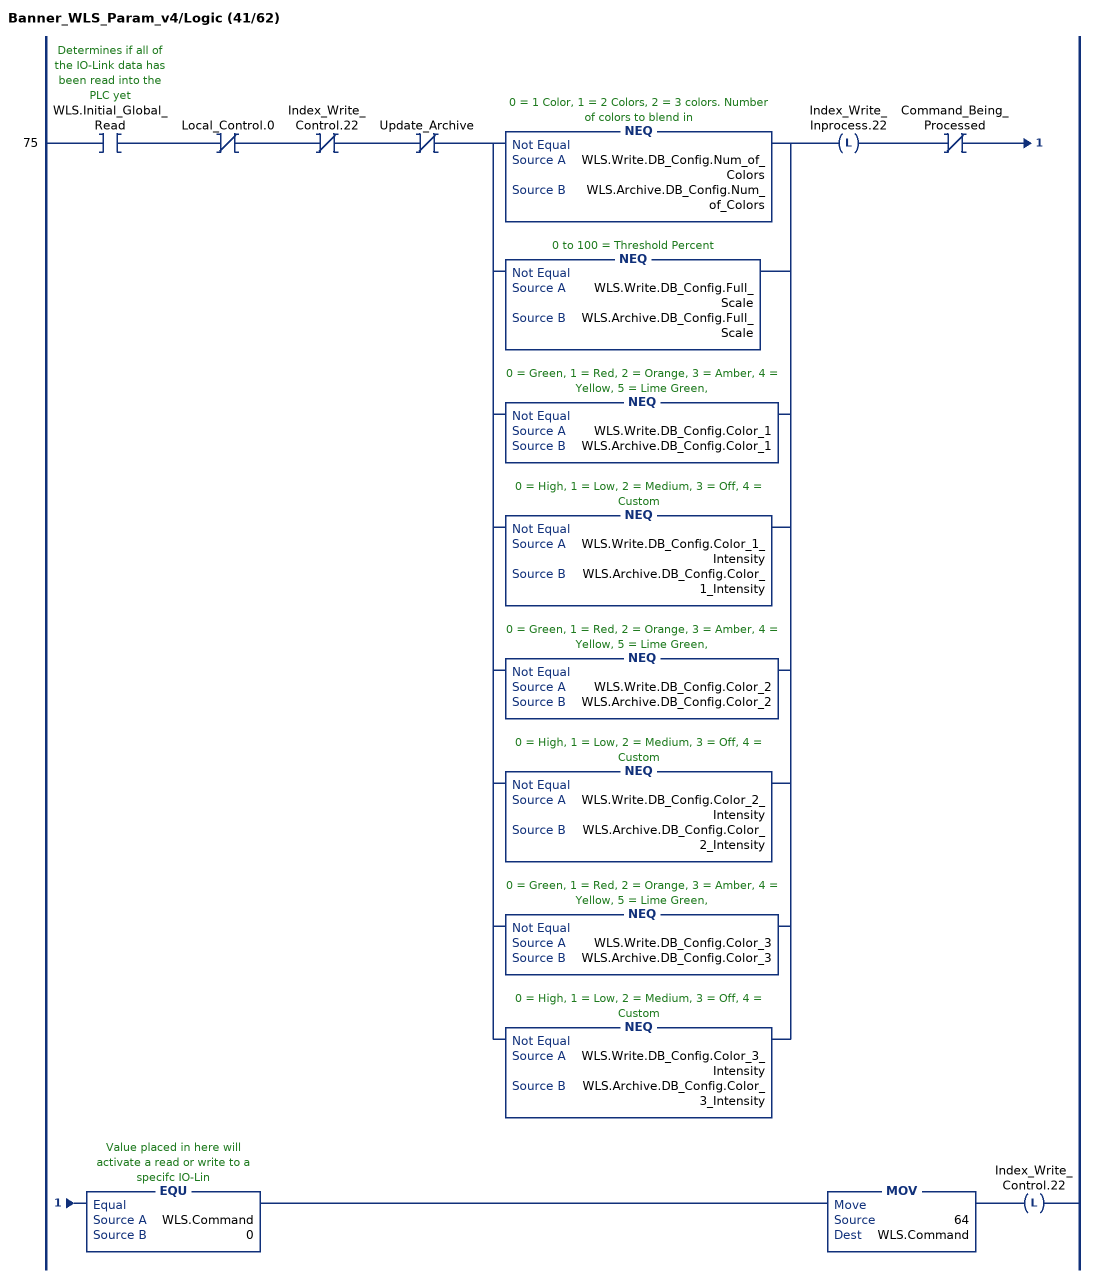
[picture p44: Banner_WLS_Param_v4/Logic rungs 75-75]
   75: XIC(WLS.Initial_Global_Read)XIO(Local_Control.0)XIO(Index_Write_Control.22)XIO(Update_Archive)[NEQ(WLS.Write.DB_Config.Num_of_Colors,WLS.Archive.DB_Config.Num_of_Colors) ,NEQ(WLS.Write.DB_Config.Full_Scale,WLS.Archive.DB_Config.Full_Scale) ,NEQ(WLS.Write.DB_Config.Color_1,WLS.Archive.DB_Config.Color_1) ,NEQ(WLS.Write.DB_Config.Color_1_Intensity,WLS.Archive.DB_Config.Color_1_Intensity) ,NEQ(WLS.Write.DB_Config.Color_2,WLS.Archive.DB_Config.Color_2) ,NEQ(WLS.Write.DB_Config.Color_2_Intensity,WLS.Archive.DB_Config.Color_2_Intensity) ,NEQ(WLS.Write.DB_Config.Color_3,WLS.Archive.DB_Config.Color_3) ,NEQ(WLS.Write.DB_Config.Color_3_Intensity,WLS.Archive.DB_Config.Color_3_Intensity) ]OTL(Index_Write_Inprocess.22)XIO(Command_Being_Processed)EQU(WLS.Command,0)MOV(64,WLS.Command)OTL(Index_Write_Control.22);
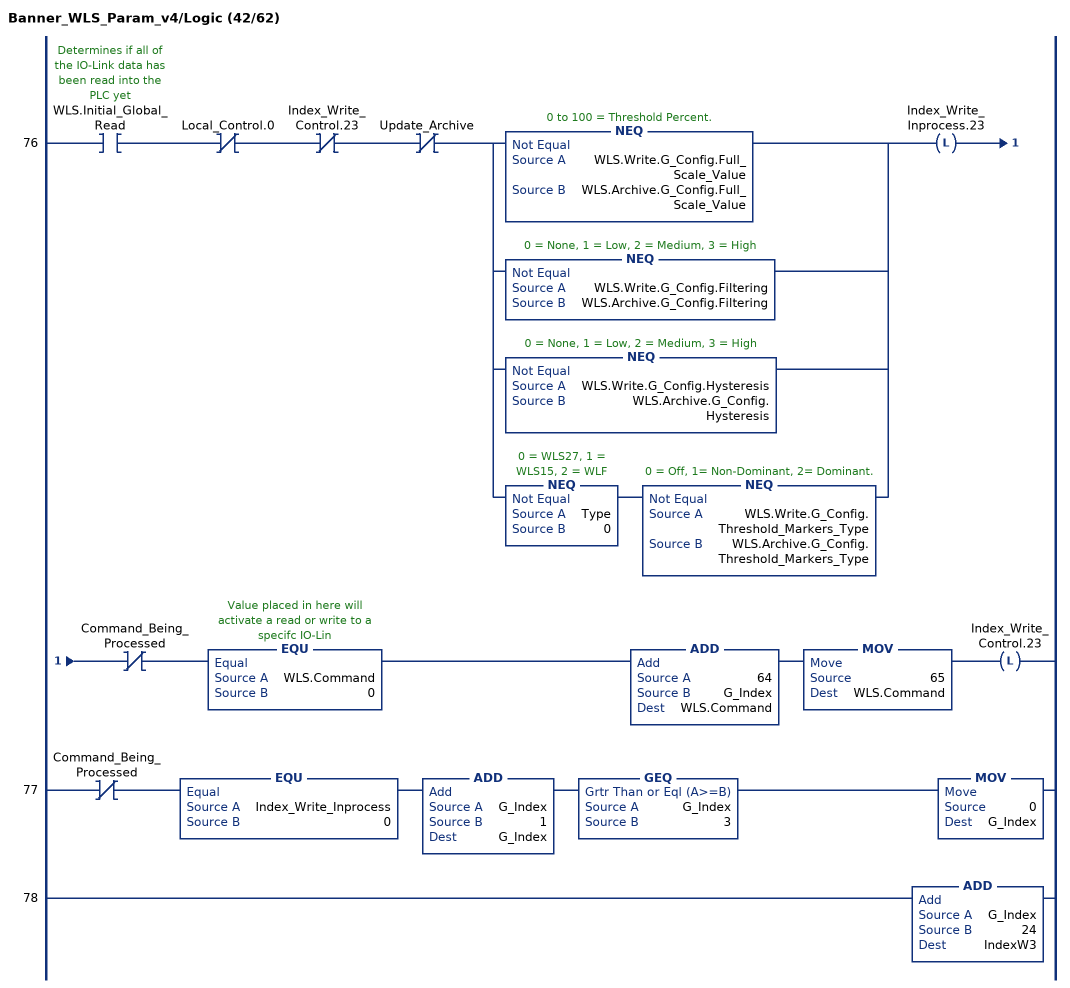
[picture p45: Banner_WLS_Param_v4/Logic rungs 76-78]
   76: XIC(WLS.Initial_Global_Read)XIO(Local_Control.0)XIO(Index_Write_Control.23)XIO(Update_Archive)[NEQ(WLS.Write.G_Config.Full_Scale_Value,WLS.Archive.G_Config.Full_Scale_Value) ,NEQ(WLS.Write.G_Config.Filtering,WLS.Archive.G_Config.Filtering) ,NEQ(WLS.Write.G_Config.Hysteresis,WLS.Archive.G_Config.Hysteresis) ,NEQ(Type,0) NEQ(WLS.Write.G_Config.Threshold_Markers_Type,WLS.Archive.G_Config.Threshold_Markers_Type) ]OTL(Index_Write_Inprocess.23)XIO(Command_Being_Processed)EQU(WLS.Command,0)ADD(64,G_Index,WLS.Command)MOV(65,WLS.Command)OTL(Index_Write_Control.23);
   77: XIO(Command_Being_Processed)EQU(Index_Write_Inprocess,0)ADD(G_Index,1,G_Index)GEQ(G_Index,3)MOV(0,G_Index);
   78: ADD(G_Index,24,IndexW3);
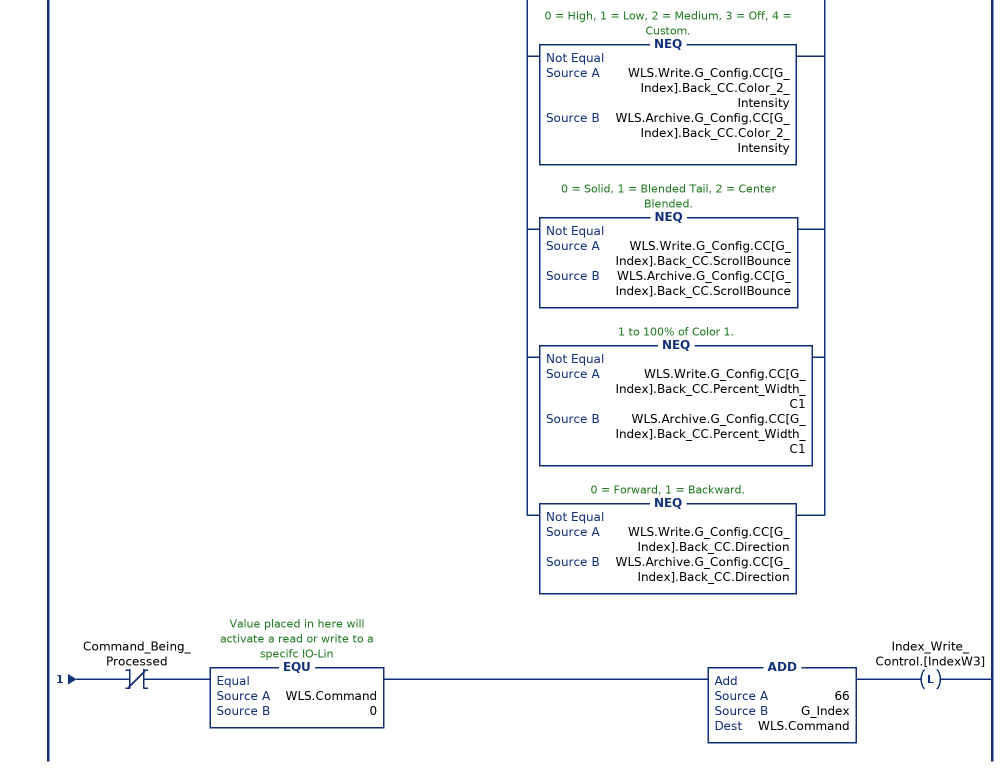
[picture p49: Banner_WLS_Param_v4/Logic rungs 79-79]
   79: XIC(WLS.Initial_Global_Read)XIO(Local_Control.0)XIO(Index_Write_Control.[IndexW3])XIO(Update_Archive)[NEQ(WLS.Write.G_Config.CC[G_Index].Threshold_Enable,WLS.Archive.G_Config.CC[G_Index].Threshold_Enable) ,NEQ(WLS.Write.G_Config.CC[G_Index].Threshold_Value_Percent,WLS.Archive.G_Config.CC[G_Index].Threshold_Value_Percent) ,NEQ(WLS.Write.G_Config.CC[G_Index].Threshold_Comparison,WLS.Archive.G_Config.CC[G_Index].Threshold_Comparison) ,NEQ(WLS.Write.G_Config.CC[G_Index].Percent_Width_of_Main_Segment,WLS.Archive.G_Config.CC[G_Index].Percent_Width_of_Main_Segment) ,NEQ(WLS.Write.G_Config.CC[G_Index].Main_CC.Animation,WLS.Archive.G_Config.CC[G_Index].Main_CC.Animation) ,NEQ(WLS.Write.G_Config.CC[G_Index].Main_CC.Color_1,WLS.Archive.G_Config.CC[G_Index].Main_CC.Color_1) ,NEQ(WLS.Write.G_Config.CC[G_Index].Main_CC.Color_1_Intensity,WLS.Archive.G_Config.CC[G_Index].Main_CC.Color_1_Intensity) ,NEQ(WLS.Write.G_Config.CC[G_Index].Main_CC.Speed,WLS.Archive.G_Config.CC[G_Index].Main_CC.Speed) ,NEQ(WLS.Write.G_Config.CC[G_Index].Main_CC.Pulse_Pattern,WLS.Archive.G_Config.CC[G_Index].Main_CC.Pulse_Pattern) ,NEQ(WLS.Write.G_Config.CC[G_Index].Main_CC.Color_2,WLS.Archive.G_Config.CC[G_Index].Main_CC.Color_2) ,NEQ(WLS.Write.G_Config.CC[G_Index].Main_CC.Color_2_Intensity,WLS.Archive.G_Config.CC[G_Index].Main_CC.Color_2_Intensity) ,NEQ(WLS.Write.G_Config.CC[G_Index].Main_CC.ScrollBounce,WLS.Archive.G_Config.CC[G_Index].Main_CC.ScrollBounce) ,NEQ(WLS.Write.G_Config.CC[G_Index].Main_CC.Percent_Width_C1,WLS.Archive.G_Config.CC[G_Index].Main_CC.Percent_Width_C1) ,NEQ(WLS.Write.G_Config.CC[G_Index].Main_CC.Direction,WLS.Archive.G_Config.CC[G_Index].Main_CC.Direction) ,NEQ(WLS.Write.G_Config.CC[G_Index].Back_CC.Animation,WLS.Archive.G_Config.CC[G_Index].Back_CC.Animation) ,NEQ(WLS.Write.G_Config.CC[G_Index].Back_CC.Color_1,WLS.Archive.G_Config.CC[G_Index].Back_CC.Color_1) ,NEQ(WLS.Write.G_Config.CC[G_Index].Back_CC.Color_1_Intensity,WLS.Archive.G_Config.CC[G_Index].Back_CC.Color_1_Intensity) ,NEQ(WLS.Write.G_Config.CC[G_Index].Back_CC.Speed,WLS.Archive.G_Config.CC[0].Back_CC.Speed) ,NEQ(WLS.Write.G_Config.CC[G_Index].Back_CC.Pulse_Pattern,WLS.Archive.G_Config.CC[G_Index].Back_CC.Pulse_Pattern) ,NEQ(WLS.Write.G_Config.CC[G_Index].Back_CC.Color_2,WLS.Archive.G_Config.CC[G_Index].Back_CC.Color_2) ,NEQ(WLS.Write.G_Config.CC[G_Index].Back_CC.Color_2_Intensity,WLS.Archive.G_Config.CC[G_Index].Back_CC.Color_2_Intensity) ,NEQ(WLS.Write.G_Config.CC[G_Index].Back_CC.ScrollBounce,WLS.Archive.G_Config.CC[G_Index].Back_CC.ScrollBounce) ,NEQ(WLS.Write.G_Config.CC[G_Index].Back_CC.Percent_Width_C1,WLS.Archive.G_Config.CC[G_Index].Back_CC.Percent_Width_C1) ,NEQ(WLS.Write.G_Config.CC[G_Index].Back_CC.Direction,WLS.Archive.G_Config.CC[G_Index].Back_CC.Direction) ]OTL(Index_Write_Inprocess.[IndexW3])XIO(Command_Being_Processed)EQU(WLS.Command,0)ADD(66,G_Index,WLS.Command)OTL(Index_Write_Control.[IndexW3]);
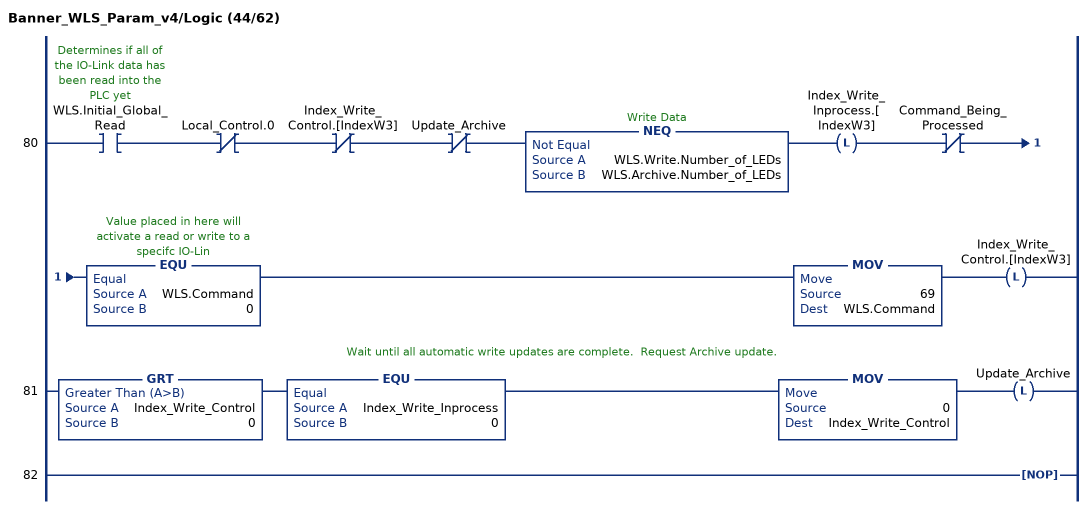
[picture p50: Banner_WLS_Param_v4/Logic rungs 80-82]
   80: XIC(WLS.Initial_Global_Read)XIO(Local_Control.0)XIO(Index_Write_Control.[IndexW3])XIO(Update_Archive)NEQ(WLS.Write.Number_of_LEDs,WLS.Archive.Number_of_LEDs)OTL(Index_Write_Inprocess.[IndexW3])XIO(Command_Being_Processed)EQU(WLS.Command,0)MOV(69,WLS.Command)OTL(Index_Write_Control.[IndexW3]);
   // Wait until all automatic write updates are complete.  Request Archive update.
   81: GRT(Index_Write_Control,0)EQU(Index_Write_Inprocess,0)MOV(0,Index_Write_Control)OTL(Update_Archive);
   82: NOP();
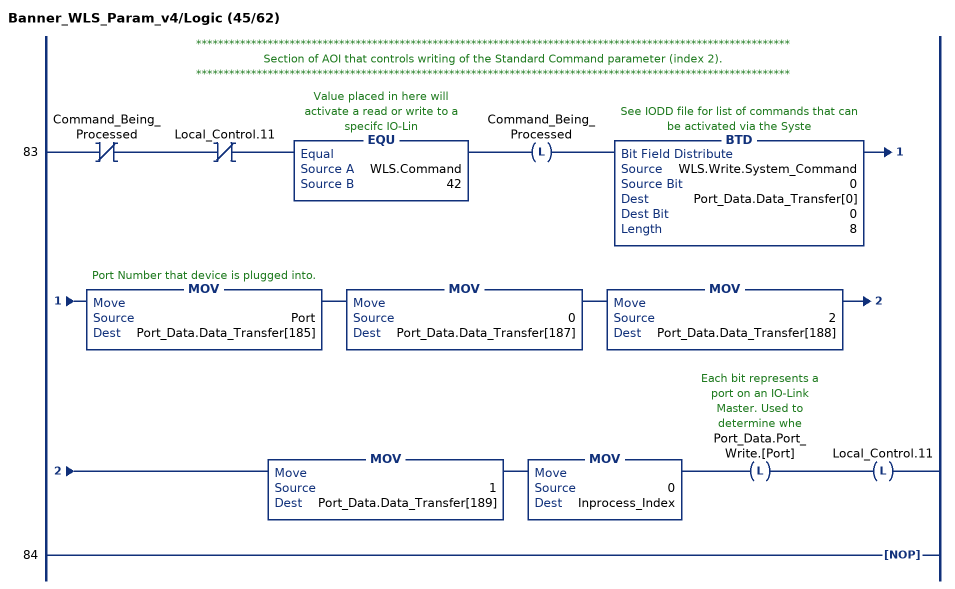
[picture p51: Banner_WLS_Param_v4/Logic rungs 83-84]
   // ************************************************************************************************************
   // Section of AOI that controls writing of the Standard Command parameter (index 2).
   // ************************************************************************************************************
   83: XIO(Command_Being_Processed)XIO(Local_Control.11)EQU(WLS.Command,42)OTL(Command_Being_Processed)BTD(WLS.Write.System_Command,0,Port_Data.Data_Transfer[0],0,8)MOV(Port,Port_Data.Data_Transfer[185])MOV(0,Port_Data.Data_Transfer[187])MOV(2,Port_Data.Data_Transfer[188])MOV(1,Port_Data.Data_Transfer[189])MOV(0,Inprocess_Index)OTL(Port_Data.Port_Write.[Port])OTL(Local_Control.11);
   84: NOP();
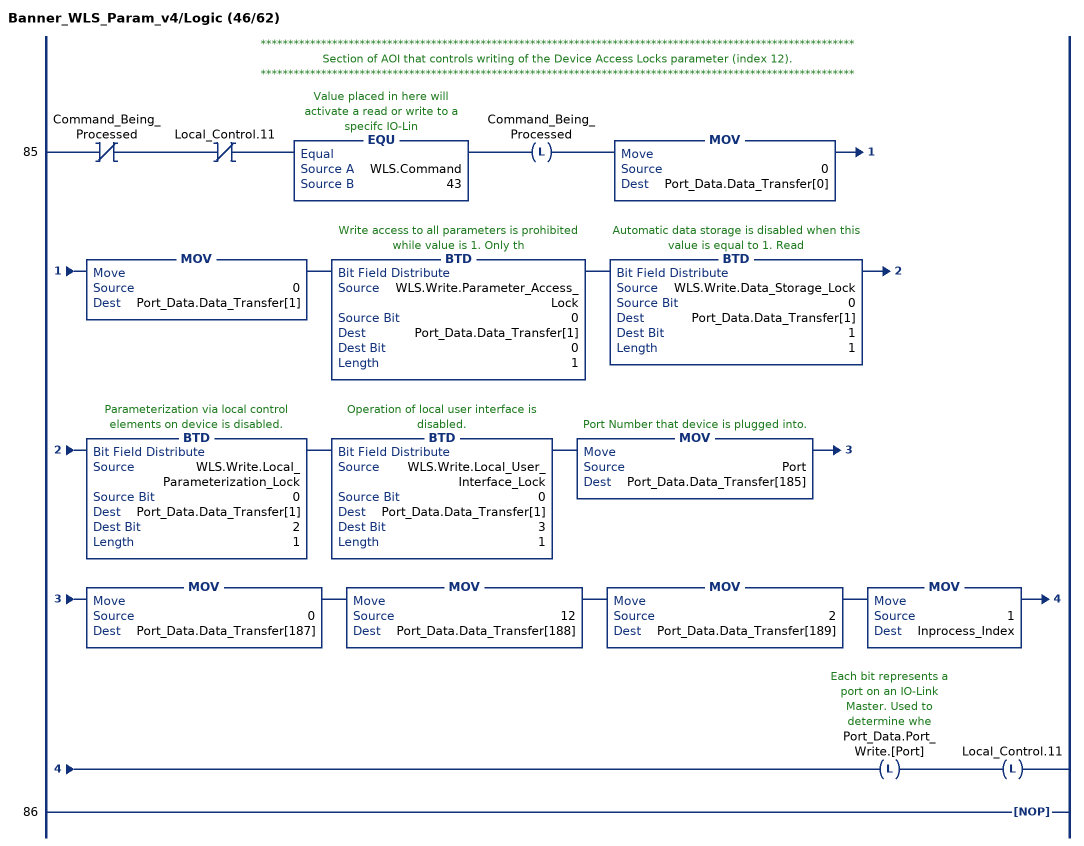
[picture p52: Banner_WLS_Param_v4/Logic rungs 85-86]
   // ************************************************************************************************************
   // Section of AOI that controls writing of the Device Access Locks parameter (index 12).
   // ************************************************************************************************************
   85: XIO(Command_Being_Processed)XIO(Local_Control.11)EQU(WLS.Command,43)OTL(Command_Being_Processed)MOV(0,Port_Data.Data_Transfer[0])MOV(0,Port_Data.Data_Transfer[1])BTD(WLS.Write.Parameter_Access_Lock,0,Port_Data.Data_Transfer[1],0,1)BTD(WLS.Write.Data_Storage_Lock,0,Port_Data.Data_Transfer[1],1,1)BTD(WLS.Write.Local_Parameterization_Lock,0,Port_Data.Data_Transfer[1],2,1)BTD(WLS.Write.Local_User_Interface_Lock,0,Port_Data.Data_Transfer[1],3,1)MOV(Port,Port_Data.Data_Transfer[185])MOV(0,Port_Data.Data_Transfer[187])MOV(12,Port_Data.Data_Transfer[188])MOV(2,Port_Data.Data_Transfer[189])MOV(1,Inprocess_Index)OTL(Port_Data.Port_Write.[Port])OTL(Local_Control.11);
   86: NOP();
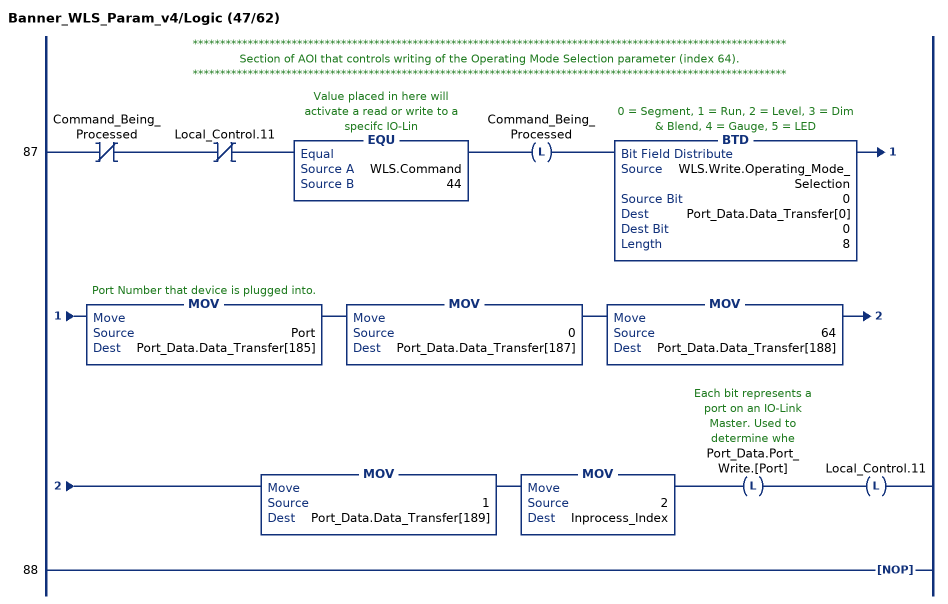
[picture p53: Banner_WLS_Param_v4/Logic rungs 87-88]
   // ************************************************************************************************************
   // Section of AOI that controls writing of the Operating Mode Selection parameter (index 64).
   // ************************************************************************************************************
   87: XIO(Command_Being_Processed)XIO(Local_Control.11)EQU(WLS.Command,44)OTL(Command_Being_Processed)BTD(WLS.Write.Operating_Mode_Selection,0,Port_Data.Data_Transfer[0],0,8)MOV(Port,Port_Data.Data_Transfer[185])MOV(0,Port_Data.Data_Transfer[187])MOV(64,Port_Data.Data_Transfer[188])MOV(1,Port_Data.Data_Transfer[189])MOV(2,Inprocess_Index)OTL(Port_Data.Port_Write.[Port])OTL(Local_Control.11);
   88: NOP();
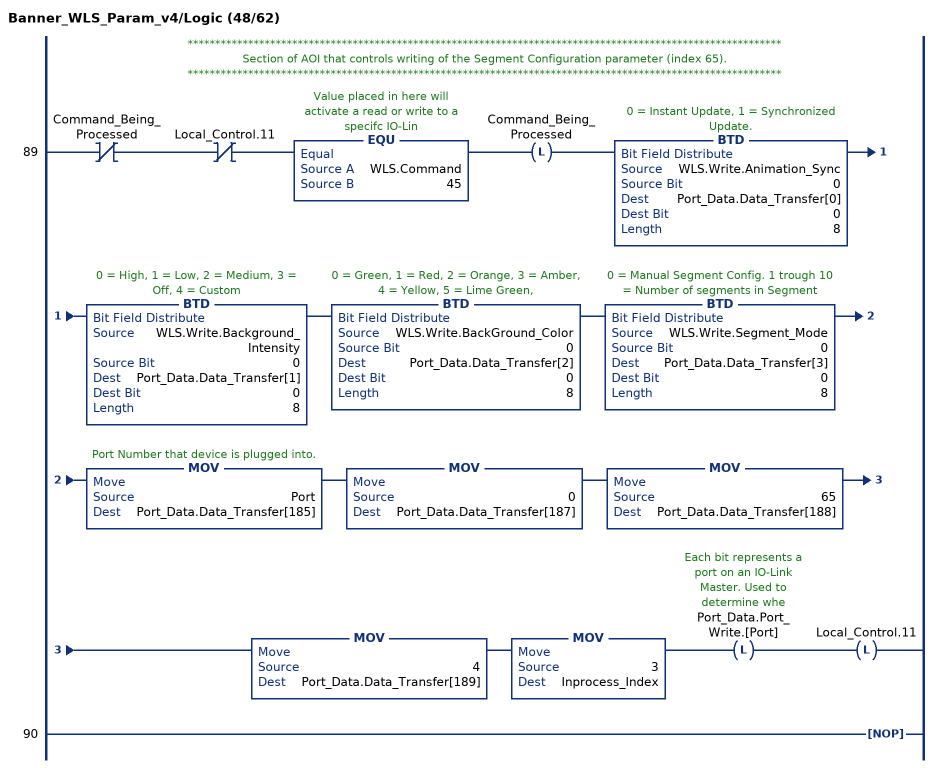
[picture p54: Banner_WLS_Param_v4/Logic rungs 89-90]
   // ************************************************************************************************************
   // Section of AOI that controls writing of the Segment Configuration parameter (index 65).
   // ************************************************************************************************************
   89: XIO(Command_Being_Processed)XIO(Local_Control.11)EQU(WLS.Command,45)OTL(Command_Being_Processed)BTD(WLS.Write.Animation_Sync,0,Port_Data.Data_Transfer[0],0,8)BTD(WLS.Write.Background_Intensity,0,Port_Data.Data_Transfer[1],0,8)BTD(WLS.Write.BackGround_Color,0,Port_Data.Data_Transfer[2],0,8)BTD(WLS.Write.Segment_Mode,0,Port_Data.Data_Transfer[3],0,8)MOV(Port,Port_Data.Data_Transfer[185])MOV(0,Port_Data.Data_Transfer[187])MOV(65,Port_Data.Data_Transfer[188])MOV(4,Port_Data.Data_Transfer[189])MOV(3,Inprocess_Index)OTL(Port_Data.Port_Write.[Port])OTL(Local_Control.11);
   90: NOP();
